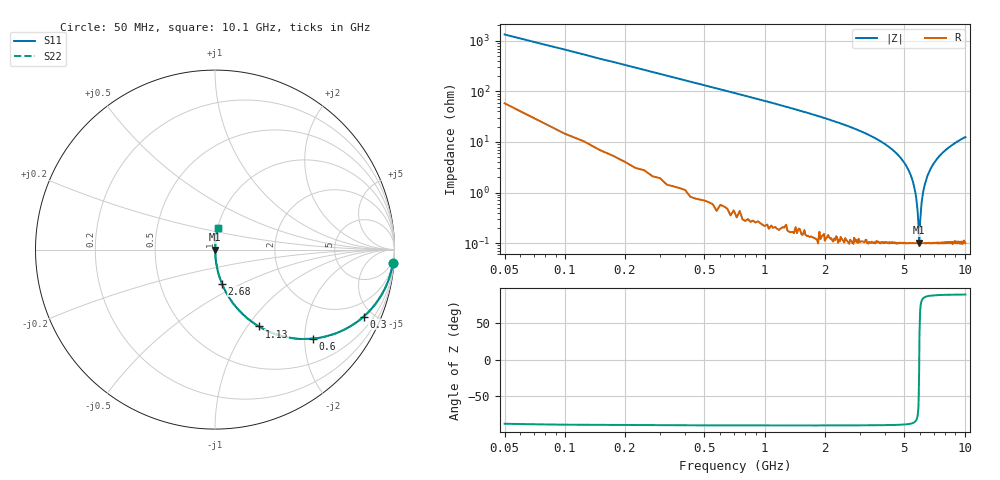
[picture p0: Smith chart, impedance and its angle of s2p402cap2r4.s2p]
! AVX Thin Film Operation		Date: April 2003
! Description: Accu-P® Series, Thin Film, SMD, RF Capacitor
! Part Number: 04025J2R4ABS
! 50 MHz  -  10.05 GHz
! Serial Measurements
# hz S db R 50
!	S11		S21		S12		S22
!	dB	Phase	dB	Phase	dB	Phase	dB	Phase
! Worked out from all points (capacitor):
!   400 points, 50 MHz to 10.1 GHz, reference 50 ohm
!   read as one part in series: C = 2.39 pF near 100 MHz
!   lowest |Z| = 103 mohm at 5.93 GHz (marker M1)
!   series resonance near 5.935 GHz, so ESL is about 300 pH
!   S11 on the Smith chart (normalised r, x): 50 MHz: 2, -26; 300 MHz: 1.04, -4.41; 600 MHz: 1.01, -2.19; 1.13 GHz: 1.00, -1.14; 2.68 GHz: 1.00, -0.39; 10.1 GHz: 1.00, +0.25
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5e7  -0.05 -4.3  -22.50 83.2  -22.50 83.2  -0.05 -4.3
1e8  -0.13 -8.6  -16.60 80.2  -16.60 80.2  -0.13 -8.6
1.5e8  -0.24 -12.7  -13.10 76.4  -13.10 76.4  -0.24 -12.7
3e8  -0.84 -24.3  -7.71 65.2  -7.71 65.2  -0.84 -24.3
6e8  -2.66 -42.3  -3.44 47.4  -3.44 47.4  -2.66 -42.3
1.13e9  -6.14 -60.2  -1.23 29.6  -1.23 29.6  -6.14 -60.2
1.73e9  -9.59 -70.4  -0.52 19.4  -0.52 19.4  -9.59 -70.4
2.68e9  -14.30 -78.5  -0.18 11.2  -0.18 11.2  -14.30 -78.5
3.4e9  -17.70 -82.1  -0.08 7.5  -0.08 7.5  -17.70 -82.1
4.38e9  -23.20 -85.2  -0.03 4.0  -0.03 4.0  -23.20 -85.2
5.08e9  -29.10 -86.4  -0.01 2.0  -0.01 2.0  -29.10 -86.4
5.48e9  -34.90 -85.8  -0.01 1.0  -0.01 1.0  -34.90 -85.8
5.68e9  -40.10 -83.7  -0.01 0.6  -0.01 0.6  -40.10 -83.7
5.83e9  -47.60 -75.9  -0.01 0.2  -0.01 0.2  -47.60 -75.9
5.93e9  -59.80 -13.5  -0.01 0.0  -0.01 0.0  -59.80 -13.5
6.05e9  -46.90 77.0  -0.01 -0.3  -0.01 -0.3  -46.90 77.0
6.2e9  -40.00 83.7  -0.01 -0.6  -0.01 -0.6  -40.00 83.7
6.45e9  -34.50 85.9  -0.01 -1.1  -0.01 -1.1  -34.50 85.9
6.75e9  -30.80 86.4  -0.01 -1.7  -0.01 -1.7  -30.80 86.4
7.5e9  -25.50 85.9  -0.02 -3.0  -0.02 -3.0  -25.50 85.9
8.43e9  -22.00 84.7  -0.04 -4.6  -0.04 -4.6  -22.00 84.7
1.01e10  -18.20 82.5  -0.07 -7.0  -0.07 -7.0  -18.20 82.5
